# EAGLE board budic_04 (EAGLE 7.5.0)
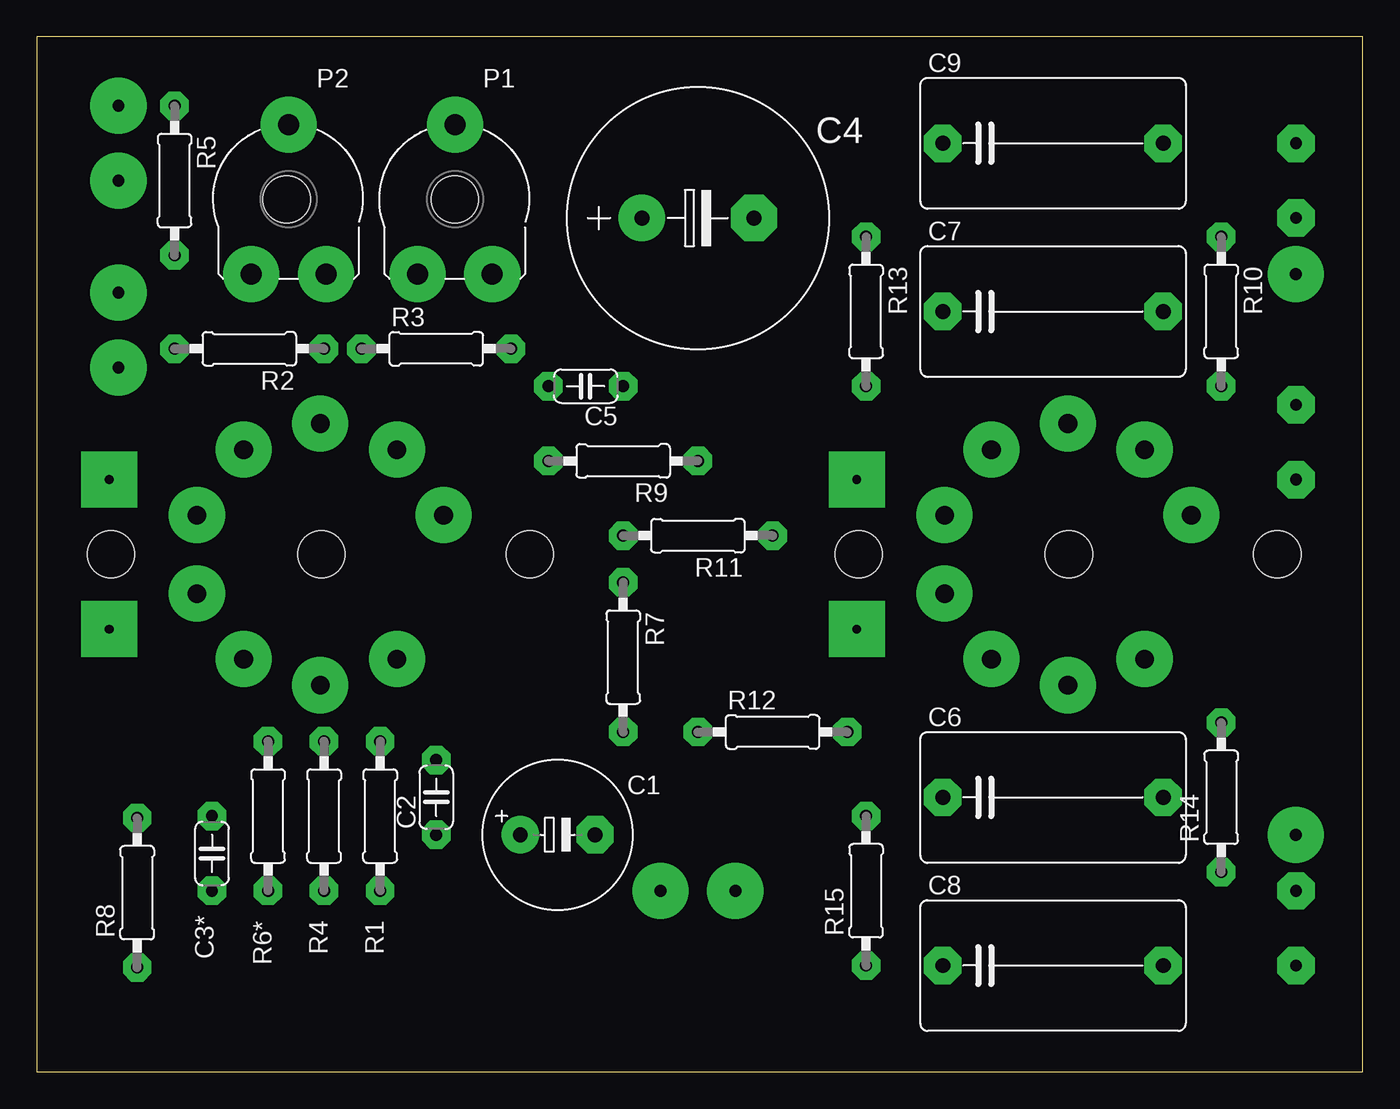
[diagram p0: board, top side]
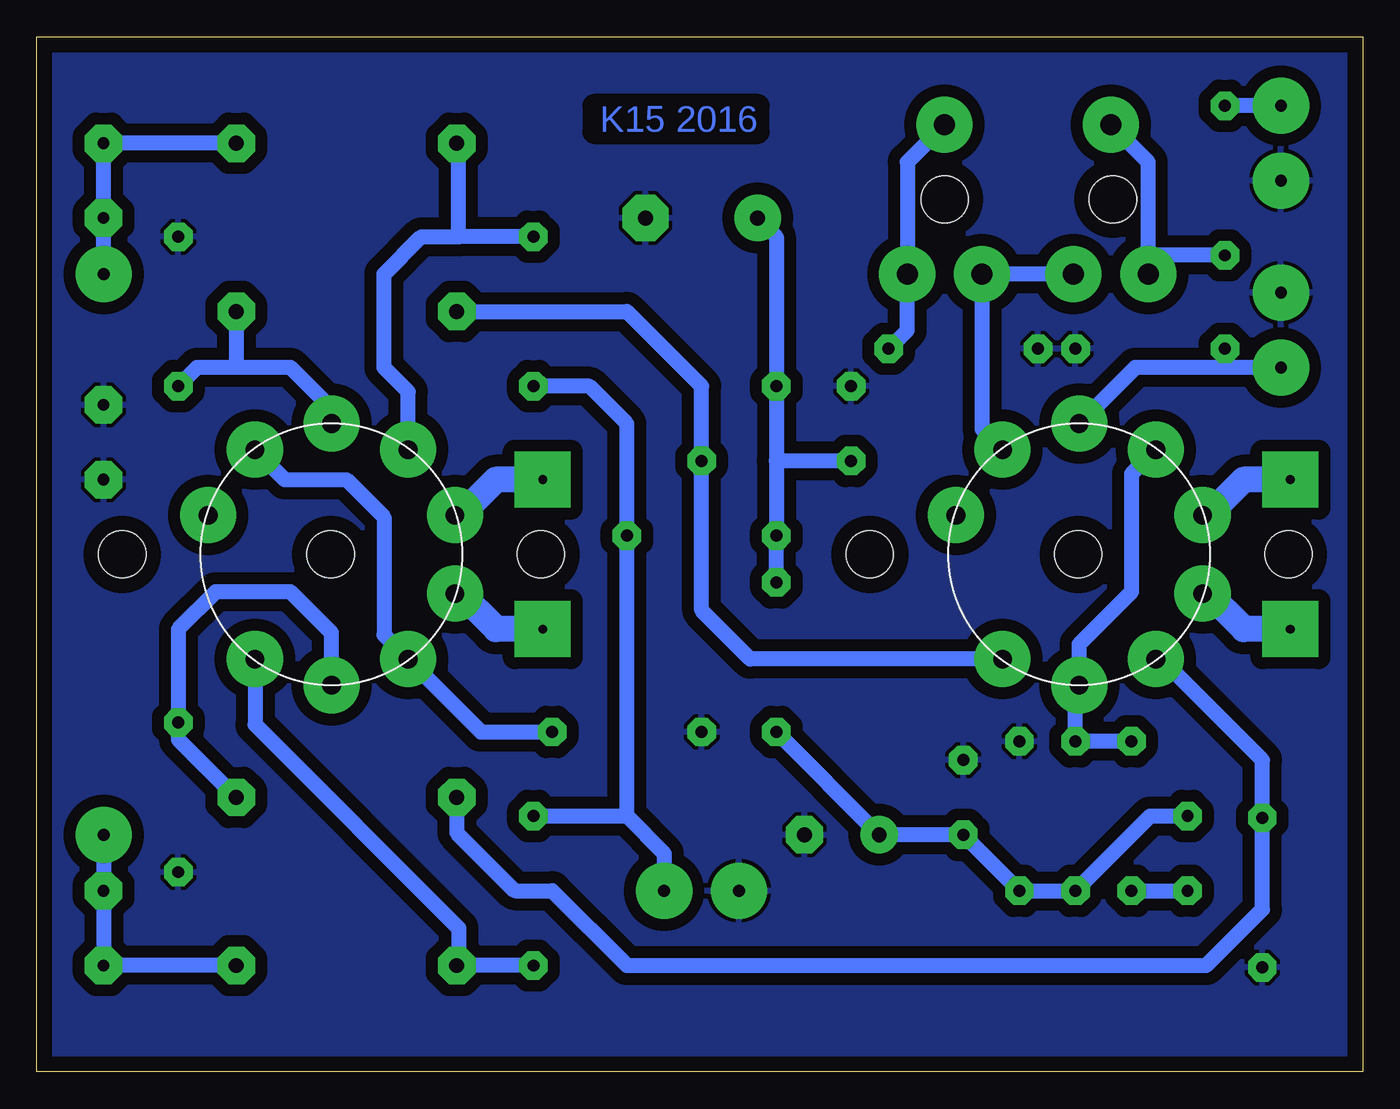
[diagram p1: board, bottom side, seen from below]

Size 90.09 x 70.34 mm. Coordinates in mm from the lower left corner, seen from the top.
Outline: 0,70.34 0,0 90.09,0 90.09,70.34 0,70.34
Copper layers (1*16): Top 0.035mm / dielectric 1.5mm / Bottom 0.035mm
Design rules "default": minimum track width 10mil, minimum drill 24mil, track to track 8mil, track to pad 8mil, pad to pad 8mil, via to via 8mil, smd to smd 8mil, copper to edge 40mil, drill to drill 8mil, minimum pad ring 10mil, minimum via ring 8mil, stop-mask expansion 4mil, vias tented up to drill 0mil, thermal gap 10mil
Holes 3.2 mm at 84.29,35.16 55.84,35.16 5.04,35.16 33.49,35.16 16.98,59.29 28.41,59.29 19.33,35.16 70.13,35.16

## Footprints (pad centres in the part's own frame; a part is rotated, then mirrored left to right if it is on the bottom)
E5-10,5 = drill 1.016 pad 2.54: + -2.54,0 | drill 1.016 pad 2.54 octagon: - 2.54,0
C050-024X044 = drill 0.813 pad 1.93 octagon: 1 -2.54,0; 2 2.54,0
E7,5-18 = drill 1.016 pad 3.15: + -3.81,0 | drill 1.016 pad 3.15 octagon: - 3.81,0
C150-091X182 = drill 1.016 pad 2.54 octagon: 1 -7.493,0; 2 7.493,0
NOVAL03 = drill 1.27 pad 3.81: P$1 7.112,-5.207; P$2 8.89,0; P$3 7.112,5.207; P$4 2.667,8.382; P$5 -2.667,8.382; P$6 -7.112,5.207; P$7 -8.89,0; P$8 -7.112,-5.207; P$9 -2.667,-8.382
PT10V = drill 1.422 pad 3.81: 1 -2.54,-5.08; 2 2.54,-5.08; 3 0,5.08
0207/10 = drill 0.813 pad 1.93 octagon: 1 -5.08,0; 2 5.08,0
TESTPIN2 = drill 0.8 pad 2.54 octagon: P$1 -2.54,0; P$2 2.54,0
PIN = drill 0.813 pad 3.81: P$1 0,0

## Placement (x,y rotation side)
C1  47u/160  [E5-10,5]  35.39,16.11 0 top
C2  1n  [C050-024X044]  27.14,18.65 90 top
C3*  100  [C050-024X044]  11.9,14.84 270 top
C4  47u/400  [E7,5-18]  44.92,58.02 0 top
C5  1n  [C050-024X044]  37.3,46.59 180 top
C6  1u/400V  [C150-091X182]  69.05,18.65 0 top
C7  1u/400V  [C150-091X182]  69.05,51.67 0 top
C8  1u/400V  [C150-091X182]  69.05,7.22 0 top
C9  1u/400V  [C150-091X182]  69.05,63.1 0 top
E1  ECC83  [NOVAL03]  19.27,35.16 270 bottom
E2  ECC82  [NOVAL03]  70.07,35.16 270 bottom
P1  1k  [PT10V]  28.41,59.29 0 top
P2  100k  [PT10V]  17.11,59.29 0 top
R1  100k  [0207/10]  23.33,17.38 270 top
R2  1M  [0207/10]  14.44,49.13 180 top
R3  820  [0207/10]  27.14,49.13 0 top
R4  120k  [0207/10]  19.52,17.38 270 top
R5  47k  [0207/10]  9.36,60.56 270 top
R6*  4k7  [0207/10]  15.71,17.38 270 top
R7  150k  [0207/10]  39.84,28.18 270 top
R8  47k  [0207/10]  6.82,12.18 90 top
R9  47k  [0207/10]  39.84,41.51 180 top
R10  1M  [0207/10]  80.48,51.67 270 top
R11  4k7  [0207/10]  44.92,36.43 180 top
R12  2k7  [0207/10]  50,23.1 0 top
R13  100k  [0207/10]  56.35,51.67 270 top
R14  1M  [0207/10]  80.48,18.65 90 top
R15  100k  [0207/10]  56.35,12.3 90 top
U$1  TESTPIN  [TESTPIN2]  85.56,60.56 90 top
U$2  TESTPIN  [TESTPIN2]  85.56,9.76 90 top
U$3  PIN  [PIN]  85.56,54.21 270 top
U$4  TESTPIN  [TESTPIN2]  85.56,42.78 90 top
U$14  PIN  [PIN]  85.56,16.11 270 top
U$38  input  [PIN]  5.55,47.86 270 top
U$40  PIN  [PIN]  42.38,12.3 270 top
U$42  PIN  [PIN]  5.55,65.64 270 top
U$58  PIN  [PIN]  5.55,60.56 270 top
U$62  PIN  [PIN]  5.55,52.94 270 top
UA  Ua  [PIN]  47.46,12.3 270 top

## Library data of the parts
C1 C2 C3* C4-C9 R1-R5 R6* R7-R15 = rcl
E1 E2 = lampy03
P1 P2 U$3 U$14 U$38 U$40 U$42 U$58 U$62 UA = LAMPY02
U$1 U$2 U$4 = lampy04

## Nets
A1: C8.1 E2.P$1 R15.1
GND: C1.- C2.2 C4.- C5.2 R1.1 R2.1 R3.1 R8.1 R10.1 R12.1 R14.1 U$4.P$1 U$4.P$2 U$40.P$1 U$58.P$1 U$62.P$1
N$1: C9.2 U$1.P$1 U$1.P$2 U$3.P$1
N$2: E1.P$2 E1.P$6 R4.1 R6*.1
N$3: C8.2 U$2.P$1 U$2.P$2 U$14.P$1
N$4: C4.+ C5.1 R7.1 R9.2 R11.2
N$5: P1.2 P1.3 R3.2
N$9: E1.P$7 R2.2 U$38.P$1
N$10: E1.P$8 P1.1 P2.2
N$11: C3*.2 R6*.2
N$14: C7.1 E1.P$1 R9.1
N$15: C1.+ C2.1 C3*.1 R1.2 R4.2 R7.2
N$18: E2.P$3 E2.P$8 R12.2
N$19: R11.1 R13.2 R15.2 UA.P$1
N$20: C9.1 E2.P$6 R13.1
N$22: C7.2 E2.P$7 R10.2
N$30: C6.1 E1.P$3 R8.2
N$31: C6.2 E2.P$2 R14.2
N$39: P2.1 P2.3 R5.2
N$40: R5.1 U$42.P$1

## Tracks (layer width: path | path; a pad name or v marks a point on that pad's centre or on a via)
A1
  Bottom 1.016: R15.1 C8.1 61.43,7.35 61.43,9.76 75.27,23.61 E2.P$1
GND
  pour Bottom (isolate 0.813): 89.12,69.45 89.12,0.62 1.23,0.62 1.23,69.45
N$1
  Bottom 1.016: U$3.P$1 U$1.P$1 U$1.P$2 C9.2
N$2
  Bottom 1.016: R6*.1 R4.1 19.52,26.02 E1.P$2 19.27,29.07 15.71,32.62 15.71,40.62 E1.P$6
N$3
  Bottom 1.016: U$14.P$1 U$2.P$2 U$2.P$1 C8.2
N$4
  Bottom 1.016: R7.1 R11.2 | R11.2 | C4.+ 39.84,56.75 C5.1 39.84,41.51 | 39.84,41.51 R11.2 | R9.2 39.84,41.51
N$5
  Bottom 1.016: P1.3 30.95,61.83 P1.2 30.95,50.4 R3.2
N$7  (via drill 0.6 pad 3.81)
  Bottom 1.778: v4.92,40.24 8.09,40.24 10.63,37.7
N$8  (via drill 0.6 pad 3.81)
  Bottom 1.778: v4.92,30.08 8.09,30.08 10.63,32.62
N$9
  Bottom 1.016: E1.P$7 15.46,47.86 9.36,47.86 | U$38.P$1 9.36,47.86 | R2.2 9.36,47.86
N$10
  Bottom 1.016: P2.2 P1.1 25.87,43.67 E1.P$8
N$11
  Bottom 1.016: R6*.2 15.63,12.3 C3*.2
N$12  (via drill 0.6 pad 3.81)
  Bottom 1.778: v55.71,40.24 58.89,40.24 61.43,37.7
N$13  (via drill 0.6 pad 3.81)
  Bottom 1.778: v55.71,30.08 58.89,30.08 61.43,32.62
N$14
  Bottom 1.016: E1.P$1 41.62,28.05 44.92,31.35 R9.1 44.92,46.59 50,51.67 C7.1
N$15
  Bottom 1.016: C3*.1 14.44,17.38 R4.2 R1.2 C2.1 C1.+ R7.2
N$18
  Bottom 1.016: R12.2 59.91,23.1 E2.P$3 66.51,29.7 66.51,37.7 69.05,40.24 73.24,40.24 E2.P$8
N$19
  Bottom 1.016: 50,17.38 R11.1 50,44.05 52.54,46.59 R13.2 | UA.P$1 47.46,14.84 50,17.38 | R15.2 50,17.38
N$20
  Bottom 1.016: 61.43,56.75 61.43,62.98 C9.1 | R13.1 61.43,56.75 | E2.P$6 64.86,46.21 66.51,47.86 66.51,54.21 63.97,56.75 61.43,56.75
N$22
  Bottom 1.016: E2.P$7 70.07,45.07 72.86,47.86 76.67,47.86 | 76.67,47.86 79.21,47.86 R10.2 | C7.2 76.54,47.99 76.67,47.86
N$30
  Bottom 1.016: C6.1 61.56,16.24 57.62,12.3 55.08,12.3 50,7.22 10.63,7.22 6.82,11.03 R8.2 6.82,21.19 13.68,28.05 E1.P$3
N$31
  Bottom 1.016: E2.P$2 70.07,29.83 72.86,32.62 77.94,32.62 80.48,30.08 R14.2 80.48,22.59 C6.2
N$39
  Bottom 1.016: P2.1 14.57,55.48 | 14.57,55.48 14.57,61.83 P2.3 | R5.2 14.57,55.48
N$40
  Bottom 1.016: U$42.P$1 R5.1

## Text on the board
Bottom: K15 2016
